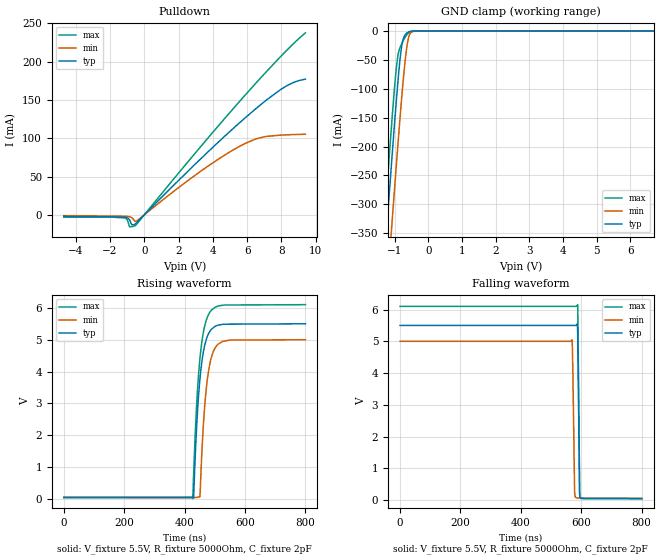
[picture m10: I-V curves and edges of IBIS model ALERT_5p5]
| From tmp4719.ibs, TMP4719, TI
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|   Model
[Model]   ALERT_5p5
Model_type   Open_drain
Polarity   Non-Inverting
Vmeas = 2.75
Vref = 5.5
Cref = 2pF
Rref = 5000
|   typ   min   max
C_comp   1.37pF   1.35pF   1.40pF
[Voltage Range]   5.5   5   6.1
[Temperature Range]   25   125   -40
[Pullup Reference]   5.5   5   6.1
[Pulldown Reference]   -0   0   0
[Power Clamp Reference]   5.5   5   6.1
[GND Clamp Reference]   0   0   0
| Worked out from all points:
|   slope of the pulldown table from 0 to 0.825 V, typ, clamps not added: 44.1 ohm
|   GND clamp passes 1 mA (typ) near -0.56 V on its own axis
|   falling waveform, V_fixture 5.5V, R_fixture 5000Ohm, C_fixture 2pF: 20-80 % time 4.17ns typ, 4.62ns min, 3.8ns max; typ from 5.5 V to 0.048 V
|   rising waveform, V_fixture 5.5V, R_fixture 5000Ohm, C_fixture 2pF: 20-80 % time 24.3ns typ, 24.1ns min, 24.6ns max; typ from 0.048 V to 5.5 V
[Pulldown]
|   Voltage   I(typ)   I(min)   I(max)
-4.7V     -2.187mA   -1.062mA   -3.034mA
-1.175V   -3.173mA   -1.862mA   -3.975mA
-1.006V   -3.881mA   -2.114mA   -6.266mA
-850.7mV  -6.924mA   -2.61mA    -15.6mA
-709.7mV  -13.13mA   -4.081mA   -15.31mA
-512.3mV  -11.49mA   -8.472mA   -13.77mA
3.238V    71.93mA    56.04mA    87.65mA
5.748V    123.9mA    91.61mA    152.8mA
7.003V    147.6mA    101.9mA    183.9mA
7.99V     164mA      104.1mA    207.4mA
8.723V    172.9mA    104.7mA    223.8mA
9.4V      177.1mA    105.2mA    237.5mA
[GND Clamp]
|   Voltage   I(typ)   I(min)   I(max)
-4.7V     -3.274A    -3.373A    -3.222A
-1.344V   -430.2mA   -544.9mA   -364.2mA
-1.161V   -281.8mA   -396.7mA   -215.8mA
-1.076V   -215mA     -329.4mA   -150mA
-949.4mV  -119.1mA   -230.7mA   -63.24mA
-893mV    -80.21mA   -188.1mA   -39.04mA
-822.5mV  -39.25mA   -136.7mA   -26.14mA
-766.1mV  -17.99mA   -97.91mA   -19.06mA
-695.6mV  -7.06mA    -54.76mA   -11.33mA
-568.7mV  -1.125mA   -7.768mA   -2.125mA
-314.9mV  -306.1nA   -10.59uA   -44.76nA
9.4V      0A         0A         0A
[Ramp]
R_load = 5000
|   typ   min   max
dV/dt_r   3.27129/2.42901e-08   2.9676/2.40284e-08   3.63359/2.46648e-08
dV/dt_f   3.27129/4.16529e-09   2.9676/4.62034e-09   3.63359/3.80402e-09
[Falling Waveform]
V_fixture = 5.5V
V_fixture_min = 5V
V_fixture_max = 6.1V
R_fixture = 5000Ohm
C_fixture = 2pF
|   Time   V(typ)   V(min)   V(max)
0s        5.5V       5V         6.1V
569.2ns   5.5V       5.046V     6.1V
571.5ns   5.5V       4.35V      6.1V
578.2ns   5.5V       243.4mV    6.1V
587ns     5.549V     67.54mV    6.126V
587.9ns   5.3V       66.91mV    6.154V
589ns     4.546V     66.1mV     5.584V
594.3ns   368.1mV    62.32mV    515.9mV
595.6ns   95.98mV    61.4mV     69.11mV
800ns     47.85mV    53.99mV    44.02mV
[Rising Waveform]
V_fixture = 5.5V
V_fixture_min = 5V
V_fixture_max = 6.1V
R_fixture = 5000Ohm
C_fixture = 2pF
|   Time   V(typ)   V(min)   V(max)
0s        47.85mV    53.99mV    44.02mV
427.2ns   54.76mV    49.44mV    10.39mV
429.9ns   39.01mV    49.41mV    745.8mV
438.5ns   2V         49.32mV    2.697V
449.9ns   3.668V     68.44mV    4.319V
465.3ns   4.768V     2.748V     5.38V
482.4ns   5.241V     4.177V     5.844V
498.3ns   5.399V     4.694V     5.997V
525.6ns   5.481V     4.945V     6.08V
800ns     5.5V       5V         6.1V
